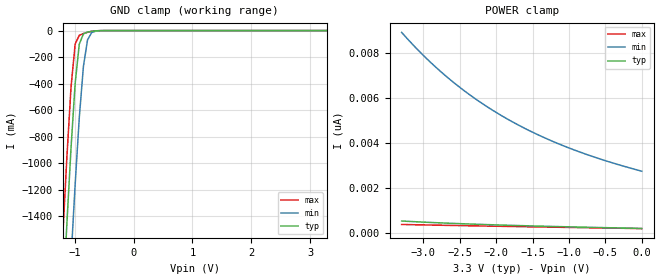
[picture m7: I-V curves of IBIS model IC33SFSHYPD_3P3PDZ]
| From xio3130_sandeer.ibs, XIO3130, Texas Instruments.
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|   Model IC33SFSHYPD_3P3PDZ
[Model]   IC33SFSHYPD_3P3PDZ
Model_type   Input
Polarity   Non-Inverting
Vinl =   0.9900V
Vinh =   2.3100V
C_comp   2.0300pF   2.1210pF   2.0450pF
[Model Spec]
|   typ   min   max
Vinh   2.31V   2.10V   2.52V
Vinl   0.99V   0.90V   1.08V
[Temperature Range]   25.0000   0.1250k   -40.0000
[Voltage Range]   3.3000V   3.0000V   3.6000V
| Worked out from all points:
|   GND clamp passes 1 mA (typ) near -0.59 V on its own axis
| (Vdd votage range)   1.50V   1.35V   1.65V
| (Process strength)   nominal   weak   strong
[GND_clamp]
| voltage   I(typ)   I(min)   I(max)
-3.3V     -22.44A    -23.23A    -22.01A
-1.2V     -2.062A    -2.938A    -1.55A
-1.13V    -1.453A    -2.319A    -952.1mA
-1.06V    -884.3mA   -1.722A    -427mA
-990mV    -399.1mA   -1.159A    -102.3mA
-920mV    -102mA     -657.3mA   -35.65mA
-850mV    -24.65mA   -270.7mA   -22.38mA
-780mV    -11.46mA   -70.03mA   -12.94mA
-710mV    -5.643mA   -15.3mA    -5.841mA
-640mV    -2.142mA   -4.304mA   -1.755mA
3.28V     186pA      2.995nA    161.1pA
[POWER_clamp]
| voltage   I(typ)   I(min)   I(max)
-3.3V     521.2pA    8.931nA    366.6pA
-3V       471.7pA    7.9nA      346.8pA
-2.85V    449.5pA    7.437nA    337.8pA
-2.65V    422.2pA    6.87nA     325.4pA
-2.3V     379.6pA    5.999nA    305.1pA
-2.1V     358pA      5.564nA    294.1pA
-1.9V     337.5pA    5.168nA    282.9pA
-1.5V     300.9pA    4.48nA     261.4pA
-1.05V    264.2pA    3.842nA    237.5pA
-550mV    227.7pA    3.263nA    211.3pA
0V        188.1pA    2.741nA    180pA
